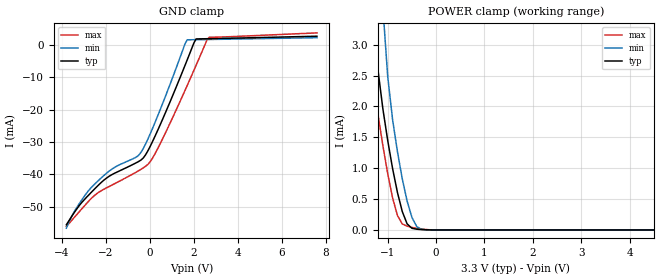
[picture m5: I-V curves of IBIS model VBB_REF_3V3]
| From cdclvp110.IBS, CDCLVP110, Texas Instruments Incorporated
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|   Reference Voltage Model for 3.3V VCC range   |
[Model]   VBB_REF_3V3
Model_type   Terminator
| Signals   VBB
| variable   typ   min   max
C_comp   0.5pF   NA   NA
[Temperature Range]   40C   110C   -40C
[Voltage range]   3.3V   3.0V   3.8V
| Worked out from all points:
|   POWER clamp passes 1 mA (typ) near -0.90 V on its own axis
[POWER Clamp]
|   40C:3.3V:nominal   110C:3.0V:weak   -40C:3.8V:strong
|  Voltage   I(typ)   I(min)   I(max)
-3.8V     128.3mA    143.1mA    114.5mA
-1.5V     6.443mA    10.41mA    3.784mA
-1.4V     4.89mA     8.555mA    2.995mA
-1.3V     3.535mA    6.761mA    2.402mA
-1.1V     1.955mA    3.582mA    1.359mA
-900mV    992.8uA    1.784mA    519.3uA
-800mV    607.8uA    1.268mA    233.8uA
-600mV    98.84uA    467.7uA    60.85uA
-500mV    26.83uA    202.8uA    41.22uA
-400mV    12.21uA    53.76uA    26.13uA
-200mV    2.935uA    2.064uA    6.782uA
7.6V      0A         0A         0A
[GND Clamp]
|   40C:3.3V:nominal   110C:3.0V:weak   -40C:3.8:strong
|  Voltage   I(typ)   I(min)   I(max)
-3.8V     -55.65mA   -56.69mA   -56.2mA
-3.3V     -50.5mA    -50.04mA   -52.29mA
-2.6V     -45.15mA   -43.65mA   -47.07mA
-1.8V     -40.41mA   -38.77mA   -43.62mA
-400mV    -35.58mA   -33.18mA   -38.45mA
-100mV    -32.87mA   -29.26mA   -37.01mA
200mV     -28.73mA   -24.53mA   -34.08mA
1.7V      -4.58mA    1.594mA    -12.52mA
2.1V      1.868mA    1.636mA    -6.325mA
2.6V      1.93mA     1.686mA    1.57mA
2.7V      1.942mA    1.696mA    2.368mA
7.6V      2.708mA    2.253mA    3.734mA
